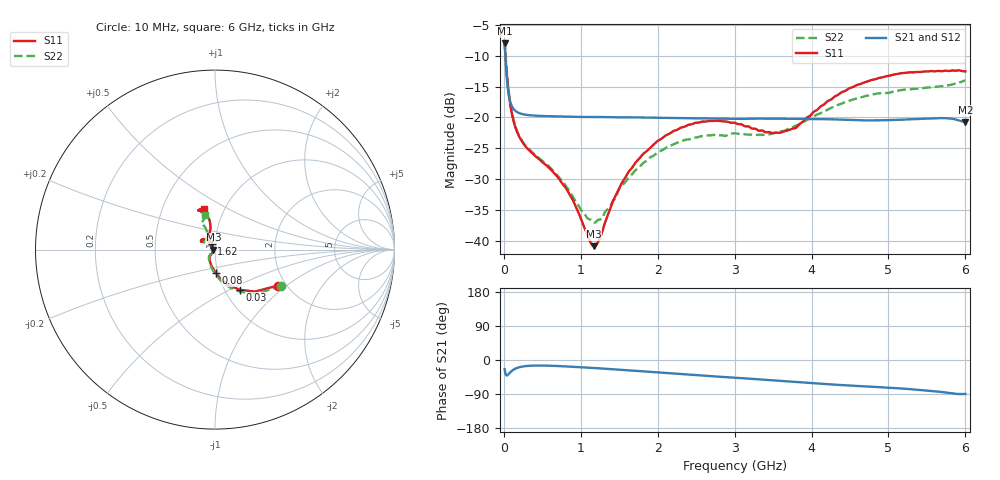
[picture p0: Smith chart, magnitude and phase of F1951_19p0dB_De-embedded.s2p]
! Integrated Device Technology
! Corporate Headquarters
! 6024 Silver Creek Valley Road
! San Jose, CA 95138  USA
! Phone:  1-408-284-8200
! Toll Free:  1-800-223-1366
! Webpage:  http://www.idt.com/
! Timing and RF Division
! 515 Groton Road, Suite 102
! Westford, MA 01886-6024
! Device:  F1951
! Description: 6-bit 0.5 dB Digital Step Attenuator
! Frequency:  100.0 -  4000.00 MHz
! Package:  4x4 mm Thin QFN Plastic Package: 24 pin
! Ports:  2 RF, 6 DC
!  Pin  1  = NC
!  Pin  2  = RF1  =  Port 1
!  Pin  3  = GND
!  Pin  4  = NC
!  Pin  5  = Serial Data Out (SDO)
!  Pin  6  = NC
!  Pin  7  = Reset Bar ( RSTb)
!  Pin  8  = Clock (CLK)
!  Pin  9  = Chip Select Bar (CSb)
!  Pin 10  = NC
!  Pin 11  = Serial Data In (SDI)
!  Pin 12  = NC
!  Pin 13  = NC
!  Pin 14  = VDD
!  Pin 15  = NC
!  Pin 16  = GND
!  Pin 17  = RF2  =  Port 2
!  Pin 18  = NC
!  Pin 19  = GND
!  Pin 20  = GND
!  Pin 21  = GND
!  Pin 22  = GND
!  Pin 23  = GND
!  Pin 24  = GND
! State:  38
! Atten State:  19.0 dB
! Voltage:  +3.30 Volts
! Current:  0.477 mA
! Data:  The device was measured on a F195X evaluation board which has
!  individual transmission lines to the RF pins.  Data was collected
!  de-embedded using a Automatic Fixture Removal [AFR] (Keysight Technologies).
!  The reference plane is the edge of the package pin.
! Misc:  Lot Code  1225BCA
!  Action Tracker AT0399
! Date Measured:  2018-09-13
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# GHz S dB R 50
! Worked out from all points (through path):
!   600 points, 10 MHz to 6 GHz, reference 50 ohm
!   highest |S21| = -8.01 dB at 10 MHz (marker M1); lowest = -20.7 dB at 6 GHz (marker M2)
!   group delay of S21, straight-line fit = 35.6 ps
!   lowest |S11| = -40.9 dB at 1.17 GHz (marker M3), VSWR 1.02, Z = 49.1 + j0.0197 ohm
!   |S11| at or under -10 dB: 20.96 MHz to end of sweep
!   |S22| runs from -37.1 to -7.5 dB; largest |S21 - S12| = 0.00026
!   S11 on the Smith chart (normalised r, x): 10 MHz: 1.82, -0.87; 30 MHz: 1.17, -0.56; 80 MHz: 0.98, -0.26; 1.62 GHz: 0.96, +0.06; 6 GHz: 0.80, +0.39
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0.01  -7.85 -29.6  -8.01 -24.3  -8.01 -24.3  -7.52 -28.8
0.03  -11.62 -58.4  -12.23 -40.1  -12.23 -40.2  -11.26 -59.3
0.05  -14.54 -73.9  -15.11 -39.7  -15.12 -39.7  -14.27 -75.4
0.08  -17.64 -87.9  -17.31 -33.3  -17.31 -33.3  -17.42 -90.0
0.15  -21.61 -106.5  -18.94 -22.8  -18.94 -22.8  -21.45 -108.6
0.25  -24.16 -119.0  -19.49 -17.0  -19.49 -16.9  -24.07 -122.3
0.71  -29.82 -127.0  -19.84 -16.0  -19.84 -16.0  -29.62 -136.6
0.87  -32.81 -128.8  -19.88 -17.7  -19.88 -17.7  -32.28 -141.3
1.01  -36.67 -137.3  -19.92 -19.2  -19.92 -19.2  -35.09 -150.6
1.17  -40.88 178.7  -19.94 -21.1  -19.94 -21.1  -37.02 -177.1
1.27  -38.91 141.6  -19.94 -22.4  -19.94 -22.4  -36.48 162.2
1.43  -33.26 121.9  -19.97 -24.6  -19.97 -24.6  -33.35 141.6
1.62  -28.85 119.1  -19.99 -27.1  -19.99 -27.2  -29.83 132.3
2.01  -23.74 127.0  -20.06 -32.8  -20.06 -32.8  -25.58 134.1
2.49  -20.88 139.9  -20.14 -39.7  -20.14 -39.7  -23.25 141.8
3.01  -20.91 149.7  -20.22 -47.0  -20.22 -46.9  -22.58 145.5
3.58  -22.51 129.4  -20.20 -54.9  -20.20 -54.9  -22.35 128.1
3.79  -21.73 113.9  -20.25 -57.9  -20.25 -57.9  -21.36 121.1
4.01  -19.33 104.4  -20.25 -61.0  -20.25 -61.0  -19.99 115.7
4.49  -15.28 100.9  -20.41 -67.5  -20.41 -67.4  -17.30 114.1
5.01  -13.24 108.6  -20.43 -73.1  -20.43 -73.1  -16.02 116.8
6  -12.53 105.2  -20.74 -89.5  -20.74 -89.5  -13.98 105.8
